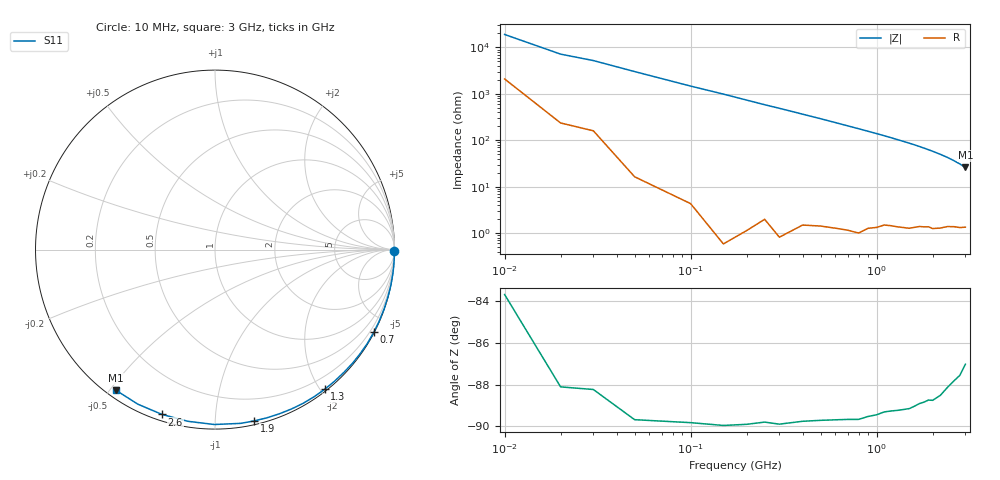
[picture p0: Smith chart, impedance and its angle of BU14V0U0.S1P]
! SIEMENS Small Signal Semiconductors
! BB833
! Si Tuning Diode in SOD323
! VR = 14 V
! S-Parameters:  April  1996
# GHz  S  MA  R  50
!  f  S11
! GHz  MAG  ANG
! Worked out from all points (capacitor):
!   31 points, 10 MHz to 3 GHz, reference 50 ohm
!   read as one part to ground: C = 1.02 pF near 10 MHz
!   lowest |Z| = 25.9 ohm at 3 GHz (marker M1)
!   S11 on the Smith chart (normalised r, x): 10 MHz: open; 700 MHz: 0.02, -4.09; 1.3 GHz: 0.03, -2.05; 1.9 GHz: 0.03, -1.25; 2.6 GHz: 0.03, -0.73; 3 GHz: 0.03, -0.52
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0.01  0.9994 -0.3
0.02  0.9995 -0.8
0.03  0.9994 -1.1
0.1  0.9998 -3.9
0.2  0.9998 -7.8
0.3  0.9997 -11.7
0.4  0.9989 -15.6
0.5  0.9984 -19.5
0.6  0.9979 -23.5
0.7  0.9974 -27.5
0.8  0.997 -31.5
0.9  0.9953 -35.5
1  0.994 -39.5
1.1  0.9918 -43.6
1.2  0.9906 -47.7
1.3  0.9896 -51.9
1.4  0.9885 -56.0
1.5  0.9873 -60.1
1.6  0.985 -64.3
1.7  0.9825 -68.6
1.8  0.9809 -72.9
1.9  0.9789 -77.2
2  0.9788 -81.5
2.2  0.9745 -90.2
2.4  0.9685 -98.9
2.6  0.9646 -107.8
2.8  0.9626 -116.5
3  0.9585 -125.2
